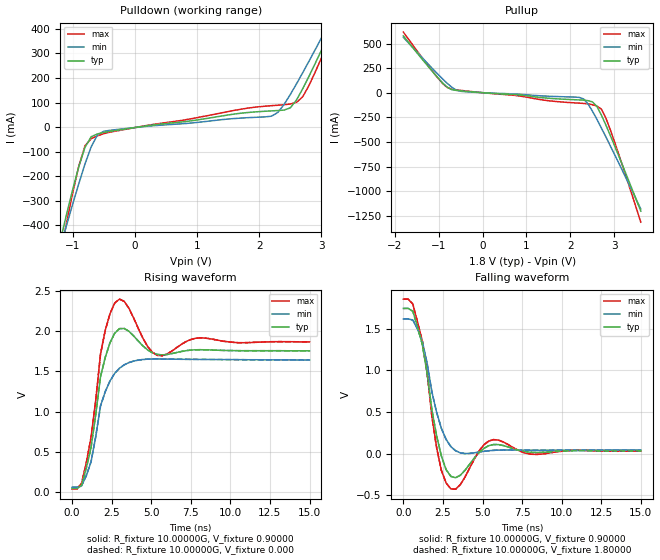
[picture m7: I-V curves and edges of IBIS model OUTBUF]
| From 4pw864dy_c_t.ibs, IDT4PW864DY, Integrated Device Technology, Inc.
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|   Model OUTBUF
[Model]   OUTBUF
Model_type   Output
Polarity   Inverting
Vmeas =  0.90000V
C_comp   6.50000pF   5.40000pF   8.10000pF
[Temperature Range]   25.00000   0.11000k   0.000
[Voltage Range]   1.80000V   1.70000V   1.90000V
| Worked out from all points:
|   slope of the pulldown table from 0 to 0.27 V, typ, clamps not added: 28.1 ohm
|   slope of the pullup table from 0 to 0.27 V, typ, clamps not added: 33.1 ohm
|   rising waveform, R_fixture 10.00000G, V_fixture 0.90000: 20-80 % time 783ps typ, 1.07ns min, 749ps max; typ from 0.047 V to 1.75 V
|   rising waveform, R_fixture 10.00000G, V_fixture 0.000: 20-80 % time 783ps typ, 1.07ns min, 749ps max; typ from 0.047 V to 1.75 V
|   falling waveform, R_fixture 10.00000G, V_fixture 0.90000: 20-80 % time 875ps typ, 1.07ns min, 831ps max; typ from 1.74 V to 0.035 V
|   falling waveform, R_fixture 10.00000G, V_fixture 1.80000: 20-80 % time 875ps typ, 1.07ns min, 831ps max; typ from 1.74 V to 0.035 V
[Pulldown]
| voltage   I(typ)   I(min)   I(max)
-1.8V     -1.128A    -1.045A    -1.344A
-1.2V     -464.6mA   -492mA     -523.8mA
-1.1V     -358.4mA   -402.5mA   -393.5mA
-900mV    -160.8mA   -229.8mA   -158.5mA
-700mV    -38.99mA   -79.32mA   -47.02mA
-500mV    -21.54mA   -16.91mA   -26.6mA
2.2V      66.18mA    44.68mA    87.4mA
2.5V      78.51mA    132.7mA    94.2mA
2.7V      156.3mA    221.7mA    123.6mA
3.1V      366.8mA    410.7mA    340.2mA
3.2V      421.6mA    459mA      400.1mA
3.6V      643.8mA    653.9mA    644.3mA
[Pullup]
| voltage   I(typ)   I(min)   I(max)
-1.8V     578.6mA    564.8mA    617.5mA
-1.1V     197.3mA    229.2mA    198mA
-800mV    57.4mA     96.09mA    53.97mA
-500mV    20.69mA    15.96mA    25.67mA
2.2V      -71.75mA   -45.81mA   -104.5mA
2.3V      -74.23mA   -62.34mA   -107.2mA
2.5V      -91.62mA   -185.8mA   -121mA
2.6V      -137.6mA   -267.6mA   -133.7mA
2.7V      -222.2mA   -353.6mA   -163.6mA
2.8V      -321.2mA   -442mA     -250.2mA
3V        -533.5mA   -623.1mA   -494.9mA
3.6V      -1.202A    -1.18A     -1.314A
[Ramp]
| variable   typ   min   max
dV/dt_r   1.02479/0.79390n   0.94624/1.13696n   1.09465/0.70536n
dV/dt_f   1.02562/0.90177n   0.94364/1.12554n   1.09424/0.84742n
R_load = 10.00000G
[Rising Waveform]
R_fixture = 10.00000G
V_fixture = 0.90000
V_fixture_min = 0.85000
V_fixture_max = 0.95000
| time   V(typ)   V(min)   V(max)
0s        47.01mV    63.93mV    40.58mV
600ps     86.83mV    82.54mV    111.3mV
1.2ns     553.6mV    379.2mV    682.6mV
1.8ns     1.433V     1.072V     1.715V
2.1ns     1.675V     1.25V      2.01V
2.7ns     1.974V     1.476V     2.348V
3ns       2.03V      1.539V     2.396V
5.4ns     1.71V      1.654V     1.698V
8.1ns     1.768V     1.648V     1.915V
15ns      1.755V     1.641V     1.865V
[Rising Waveform]
R_fixture = 10.00000G
V_fixture = 0.000
V_fixture_min = 0.000
V_fixture_max = 0.000
| time   V(typ)   V(min)   V(max)
0s        47.01mV    63.93mV    40.58mV
600ps     86.83mV    82.54mV    111.3mV
1.2ns     553.6mV    379.2mV    682.6mV
1.8ns     1.433V     1.072V     1.715V
2.1ns     1.675V     1.25V      2.01V
2.7ns     1.974V     1.476V     2.348V
3ns       2.03V      1.539V     2.396V
5.4ns     1.71V      1.654V     1.698V
8.1ns     1.768V     1.648V     1.915V
15ns      1.755V     1.641V     1.865V
[Falling Waveform]
R_fixture = 10.00000G
V_fixture = 0.90000
V_fixture_min = 0.85000
V_fixture_max = 0.95000
| time   V(typ)   V(min)   V(max)
0s        1.744V     1.617V     1.856V
600ps     1.71V      1.605V     1.797V
1.2ns     1.31V      1.346V     1.351V
2.1ns     215.7mV    498.6mV    73.85mV
2.4ns     -25.4mV    306.1mV    -198.3mV
3ns       -272.1mV   85.76mV    -422.3mV
3.6ns     -258.5mV   10.4mV     -371.4mV
5.7ns     110.4mV    40.3mV     169.4mV
8.1ns     16.7mV     41.92mV    -6.26mV
15ns      34.63mV    44.26mV    32.27mV
[Falling Waveform]
R_fixture = 10.00000G
V_fixture = 1.80000
V_fixture_min = 1.70000
V_fixture_max = 1.90000
| time   V(typ)   V(min)   V(max)
0s        1.744V     1.617V     1.856V
600ps     1.71V      1.605V     1.797V
1.2ns     1.31V      1.346V     1.351V
2.1ns     215.7mV    498.6mV    73.85mV
2.4ns     -25.4mV    306.1mV    -198.3mV
3ns       -272.1mV   85.76mV    -422.3mV
3.6ns     -258.5mV   10.4mV     -371.4mV
5.7ns     110.4mV    40.3mV     169.4mV
8.1ns     16.7mV     41.92mV    -6.26mV
15ns      34.63mV    44.26mV    32.27mV
